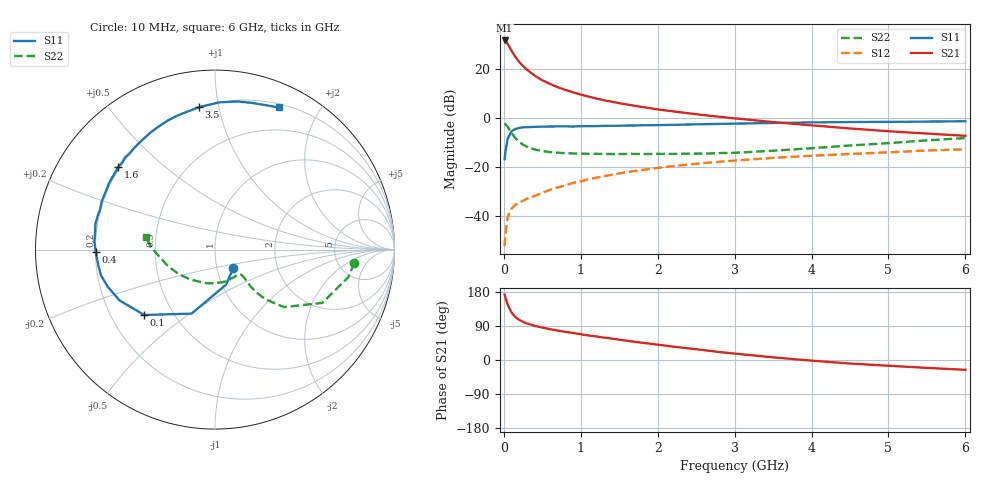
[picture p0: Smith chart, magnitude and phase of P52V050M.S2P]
! SIEMENS Small Signal Semiconductors
! BFP183
! Si NPN RF Bipolar Junction Transistor in SOT143
! VCE = 2 V  IC = 50 mA
! Common Emitter S-Parameters:  March  1996
# GHz  S  MA  R  50
!  f  S11  S21  S12  S22
! GHz  MAG  ANG  MAG  ANG  MAG  ANG  MAG  ANG
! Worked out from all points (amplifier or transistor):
!   36 points, 10 MHz to 6 GHz, reference 50 ohm
!   highest |S21| = 31.8 dB at 10 MHz (marker M1)
!   |S21| within 3 dB of that: start of sweep to 78.71 MHz
!   unconditionally stable (mu >= 1): start of sweep to 26.39 MHz; 229.2 MHz to end of sweep
!   at 250 MHz: K = 1.05, MAG = 26.2 dB, |S12| = -33.8 dB
!   at 1.4 GHz: K = 1.59, MAG = 10.5 dB, |S12| = -23.2 dB
!   at 6 GHz: K = 1.22, MAG = -0.1 dB, |S12| = -12.7 dB
!   S11 on the Smith chart (normalised r, x): 10 MHz: 1.20, -0.25; 100 MHz: 0.34, -0.35; 400 MHz: 0.20, -0.01; 1.6 GHz: 0.19, +0.36; 3.5 GHz: 0.20, +0.87; 6 GHz: 0.24, +1.52
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0.01  0.1452 -45.2  39.11 172.6  0.0024 67.8  0.7788 -5.5
0.02  0.2058 -73.0  38.39 165.4  0.0043 71.7  0.7596 -11.5
0.05  0.3799 -110.1  33.43 145.9  0.0096 62.7  0.6678 -26.4
0.1  0.5371 -137.3  24.07 125.3  0.0141 48.9  0.5005 -39.8
0.15  0.6026 -152.0  18.03 113.4  0.0169 47.7  0.3921 -44.7
0.2  0.6329 -161.0  14.21 105.9  0.0187 47.2  0.3278 -46.0
0.25  0.6506 -167.1  11.62 100.5  0.0204 49.0  0.2878 -45.9
0.3  0.6554 -171.7  9.82 96.5  0.0224 50.2  0.26 -45.3
0.4  0.6649 -178.9  7.476 90.2  0.0256 53.6  0.229 -44.1
0.5  0.6733 176.1  5.996 85.5  0.0298 56.1  0.2123 -43.6
0.6  0.6752 171.6  5.039 81.3  0.0341 57.5  0.2024 -43.7
0.7  0.6814 167.8  4.305 77.7  0.0382 59.8  0.1965 -44.4
0.9  0.6779 160.8  3.391 71.3  0.0474 60.6  0.1902 -47.3
1.1  0.6873 154.4  2.774 64.8  0.0564 60.7  0.1867 -51.0
1.3  0.6961 148.1  2.337 59.2  0.0649 60.2  0.1861 -55.9
1.6  0.7086 139.4  1.913 50.9  0.0787 58.4  0.1858 -63.5
2.2  0.7321 124.0  1.382 35.4  0.1045 52.9  0.1857 -82.4
2.8  0.7659 110.0  1.072 21.1  0.1283 46.8  0.1933 -103.7
3.5  0.798 96.6  0.834 7.0  0.1541 39.9  0.2156 -129.1
4.5  0.8348 81.4  0.617 -9.3  0.1852 29.5  0.2763 -160.1
5.5  0.8533 70.5  0.485 -20.8  0.2183 20.1  0.3526 178.6
6  0.8674 65.9  0.436 -25.9  0.2315 15.1  0.3921 169.8
